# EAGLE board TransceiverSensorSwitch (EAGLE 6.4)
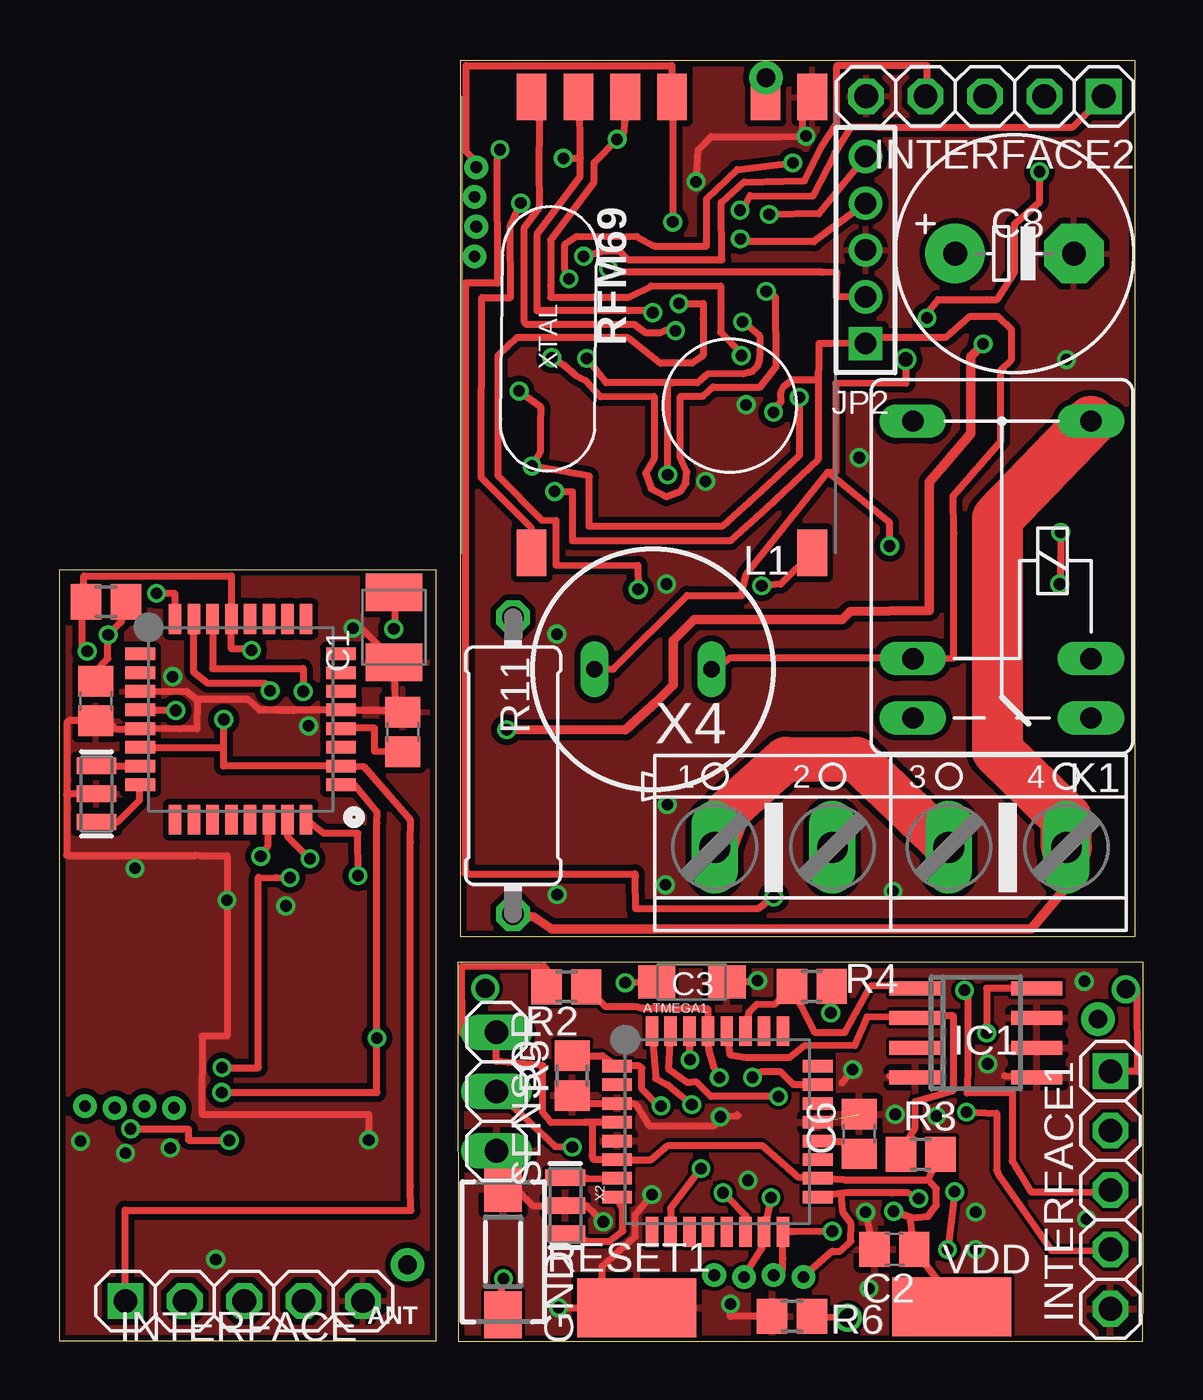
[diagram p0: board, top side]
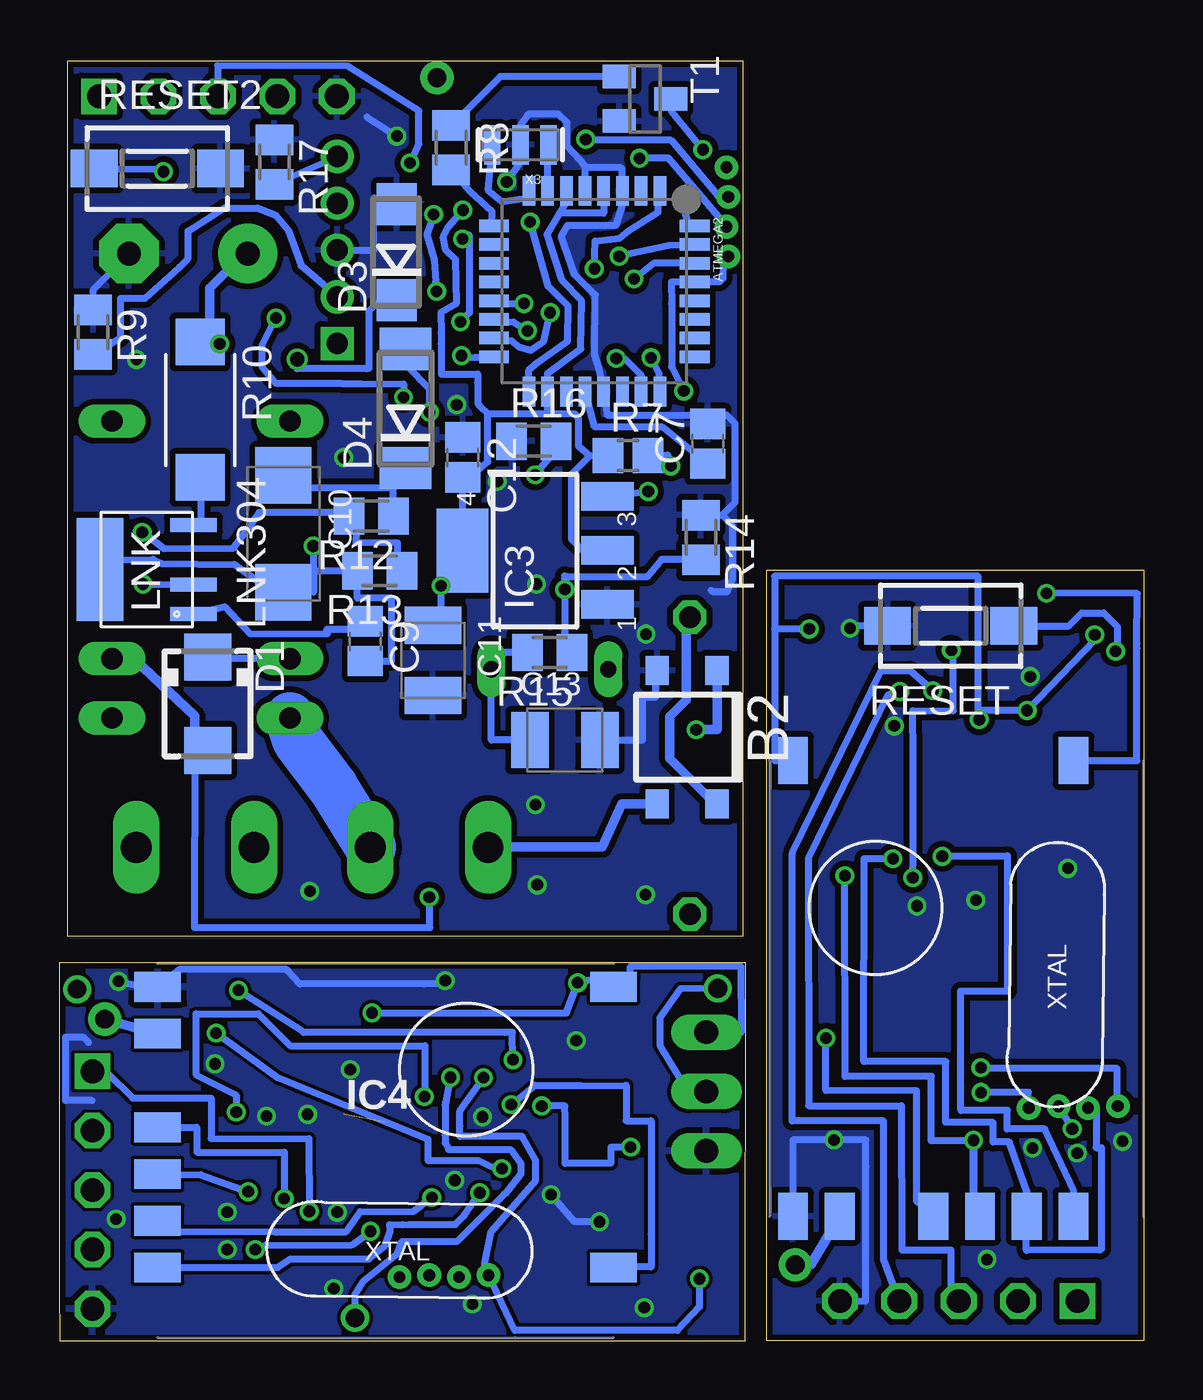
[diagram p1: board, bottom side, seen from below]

Size 46.36 x 54.77 mm. Coordinates in mm from the lower left corner, seen from the top.
Outline: 0,0.01 16.13,0.01 16.13,32.99 0,32.99 0,0.01
Outline: 17.06,0 46.34,0 46.35,2.34 46.36,15.39 46.35,16.2 17.04,16.2 17.06,0
Outline: 17.14,17.31 46.02,17.31 46.02,54.77 17.14,54.77 17.14,17.31
Copper layers (1*16): Top 0.035mm / dielectric 1.5mm / Bottom 0.035mm
Design rules "ITEADstudio_DRC": minimum track width 6mil, minimum drill 12mil, track to track 6mil, track to pad 6mil, pad to pad 6mil, via to via 6mil, smd to smd 0mil, copper to edge 10mil, drill to drill 10mil, minimum pad ring 10mil, minimum via ring 6mil, stop-mask expansion 2mil, vias tented up to drill 100mil, thermal gap 10mil
Net classes: 1 power: width 0.381 mm, clearance 0.254 mm; 2 220V: width 0.381 mm, clearance 0.508 mm

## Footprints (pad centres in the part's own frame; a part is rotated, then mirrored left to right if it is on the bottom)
TQFP32-08 = smd 1.27 x 0.533: 1 -4.293,2.8; 2 -4.293,2; 3 -4.293,1.2; 4 -4.293,0.4; 5 -4.293,-0.4; 6 -4.293,-1.2; 7 -4.293,-2; 8 -4.293,-2.8; 17 4.293,-2.8; 18 4.293,-2; 19 4.293,-1.2; 20 4.293,-0.4; 21 4.293,0.4; 22 4.293,1.2; 23 4.293,2; 24 4.293,2.8 | smd 0.533 x 1.27: 9 -2.8,-4.293; 10 -2,-4.293; 11 -1.2,-4.293; 12 -0.4,-4.293; 13 0.4,-4.293; 14 1.2,-4.293; 15 2,-4.293; 16 2.8,-4.293; 25 2.8,4.293; 26 2,4.293; 27 1.2,4.293; 28 0.4,4.293; 29 -0.4,4.293; 30 -1.2,4.293; 31 -2,4.293; 32 -2.8,4.293
TO-269AA = smd 1 x 1.25: + -1.28,-2.855; - 1.28,-2.855; AC1 -1.28,2.855; AC2 1.28,2.855
SMC_B = smd 1.6 x 2.4: + -1.5,0; - 1.5,0
C2012 = smd 1.3 x 1.5: 1 -0.85,0; 2 0.85,0
SMC_A = smd 1.6 x 1.4: + -1.5,0; - 1.5,0
E5-10,5 = drill 1.016 pad 2.54: + -2.54,0 | drill 1.016 pad 2.54 octagon: - 2.54,0
SMC_C = smd 2.4 x 2.4: + -2.5,0; - 2.5,0
SMA = smd 2 x 2: A 2,0; C -2,0
DO214AC = smd 1.8 x 1.7: A 2.05,0; C -2.05,0
DO214AA = smd 1.8 x 2.2: A 2.55,0; C -2.55,0
SMD2,54-5,08 = smd 2.54 x 5.08: 1 0,0
SO08 = smd 0.6 x 2.2: 1 -1.905,-2.6; 2 -0.635,-2.6; 3 0.635,-2.6; 4 1.905,-2.6; 5 1.905,2.6; 6 0.635,2.6; 7 -0.635,2.6; 8 -1.905,2.6
SOT223 = smd 1.219 x 2.235: 1 -2.311,-3.099; 2 0,-3.099; 3 2.311,-3.099 | smd 3.6 x 2.2: 4 0,3.099
RFM69W-MINPADS = smd 2 x 1.27: ANA 8,-5; DIO0 -11.5,5; GND 8,-7; MISO 8,1; MOSI 8,3; NSS 8,5; SCK 8,-1; VDD -11.5,-7
1X05-S = drill 1.016 square: 1 -5.08,0 | drill 1.016 octagon: 2 -2.54,0; 3 0,0; 4 2.54,0; 5 5.08,0
1X05M = drill 0.914 square: 1 -4,0 | drill 0.914: 2 -2,0; 3 0,0; 4 2,0; 5 4,0
FRS1B = drill 0.914 long: 1 0,3.81; 2 0,-3.81; O -2.54,-3.81; P 10.16,3.81; P@ 10.16,-3.81; S -2.54,3.81
BS11 = drill 0.7 long: 1 -2.5,0; 2 2.5,0
SO-8C = smd 0.6 x 2: BP -1.905,-2; D 1.905,-2; FB -0.635,-2 | smd 4.41 x 2: S 0,2
R2012 = smd 1.3 x 1.5: 1 -0.85,0; 2 0.85,0
M2012 = smd 1.3 x 1.6: 1 -0.95,0; 2 0.95,0
R2512W = smd 2 x 2.1: 1 -2.896,0; 2 2.896,0
0411/12 = drill 0.914 octagon: 1 -6.35,0; 2 6.35,0
DTSM-3 = smd 2 x 1.6: 1 -2.7,0; 2 2.7,0
1X03 = drill 1.016 long: 1 -2.54,0; 2 0,0; 3 2.54,0
SOT23 = smd 1 x 1.4: 1 -0.95,-1.1; 2 0.95,-1.1; 3 0,1.1
RFM12B-ANTENNA = drill 0.8 pad 1.422: P$1 0,0
AVRHEADER = drill 0.5: CLK 2.54,0; MISO 1.27,0.07; MOSI 0,0; VPP -1.27,0.072
RESONATOR-SMD = smd 0.7 x 1.7: 1 -1.2,0; 2 0,0; 3 1.2,0
AK500/4 = drill 1.321 long: 1 -7.518,0; 2 -2.489,0; 3 2.489,0; 4 7.518,0

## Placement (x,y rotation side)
ATMEGA1  ATMega-328  [TQFP32-08]  28.15,8.96 0 top
ATMEGA2  ATMega-328  [TQFP32-08]  23.49,44.91 270 bottom
ATMEGA328  ATMega-328  [TQFP32-08]  7.76,26.6 0 top
B2  RECT  [TO-269AA]  19.52,25.83 180 bottom
C1  100uF  [SMC_B]  14.32,30.53 90 top
C2  100nF  [C2012]  35.72,3.93 180 top
C3  100uF  [SMC_A]  27.06,15.36 0 top
C4  0.1  [C2012]  1.56,27.38 270 top
C5  0.1  [C2012]  14.69,26.05 90 top
C6  0.1  [C2012]  34.22,8.86 90 top
C7  0.1  [C2012]  18.64,38.39 90 bottom
C8  3,3uF  [E5-10,5]  40.86,46.52 0 top
C9  100nF  [C2012]  33.29,29.94 270 bottom
C10  22uF / 16 V  [SMC_C]  36.79,34.53 270 bottom
C11  100uF  [SMC_B]  30.39,29.12 270 bottom
C12  100nF  [C2012]  29.12,37.8 270 bottom
C13  100uF  [SMC_B]  24.75,25.71 0 bottom
D1  MBRA340T3  [SMA]  40.03,27.26 270 bottom
D3  ES1D  [DO214AC]  31.94,46.58 90 bottom
D4  1N4007GP  [DO214AA]  31.57,39.89 90 bottom
GND  [SMD2,54-5,08]  24.7,1.42 90 top
IC1  LM75AD  [SO08]  39.2,13.18 270 top
IC3  MC33269ST-3.3T3  [SOT223]  26.03,33.82 90 bottom
IC4  RFM69  [RFM69W-MINPADS]  34.17,8.15 180 bottom
INTERFACE  [1X05-S]  7.91,1.71 0 top
INTERFACE1  [1X05-S]  44.96,6.46 270 top
INTERFACE2  [1X05-S]  39.59,53.25 180 top
JP2  [1X05M]  34.49,46.67 90 top
K1  FRS1B  [FRS1B]  40.32,29.19 90 top
L1  680uH  [BS11]  25.4,28.74 0 top
LNK  LNK304  [SO-8C]  42.63,33.01 90 bottom
R1  10k  [R2012]  2,31.63 180 top
R2  10k  [R2012]  21.69,15.16 0 top
R3  10k  [R2012]  36.84,7.99 0 top
R4  10k  [R2012]  32.19,15.17 0 top
R5  10k  [R2012]  21.94,11.35 90 top
R6  10k  [R2012]  31.34,1.06 0 top
R7  10k  [R2012]  22.05,37.88 0 bottom
R8  1 K  [M2012]  29.62,51.05 90 bottom
R9  10K  [M2012]  44.93,43.16 270 bottom
R10  100  [R2512W]  40.35,39.85 270 bottom
R11  8,2  [0411/12]  19.41,24.62 90 top
R12  3.9 k  [M2012]  33.04,35.29 180 bottom
R13  2,05 k  [M2012]  32.68,32.95 180 bottom
R14  560  [M2012]  18.94,34.38 270 bottom
R15  470  [M2012]  25.4,29.46 180 bottom
R16  20K  [M2012]  26.09,38.5 0 bottom
R17  10K  [M2012]  37.17,50.44 270 bottom
RESET  RESET  [DTSM-3]  8.25,30.6 180 bottom
RESET1  [DTSM-3]  18.99,3.82 90 top
RESET2  RESET  [DTSM-3]  42.18,50.16 0 bottom
RFM69  RFM69  [RFM69W-MINPADS]  25.2,45.22 90 top
SENSOR  [1X03]  18.7,10.68 270 top
T1  BC846  [SOT23]  21.33,53.14 270 bottom
U$1  RFM12B_ANTENNA  [RFM12B-ANTENNA]  14.9,3.26 0 top
U$2  AVRHEADERDIP  [AVRHEADER]  2.38,9.97 0 top
U$3  RFM12B_ANTENNA  [RFM12B-ANTENNA]  44.43,13.77 0 top
U$4  AVRHEADERDIP  [AVRHEADER]  29.28,2.74 0 top
U$5  RFM69  [RFM69W-MINPADS]  8,13.33 270 bottom
U$6  RFM12B_ANTENNA  [RFM12B-ANTENNA]  30.22,54.04 0 top
U$7  AVRHEADERDIP  [AVRHEADER]  17.84,47.67 90 top
VDD  [SMD2,54-5,08]  38.17,1.47 90 top
X1  16 MHz  [RESONATOR-SMD]  1.6,23.41 270 top
X2  16 MHz  [RESONATOR-SMD]  21.65,5.8 270 top
X3  16 MHz  [RESONATOR-SMD]  26.66,51.17 180 bottom
X4  [AK500/4]  35.56,21.12 0 top

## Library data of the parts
ATMEGA1 ATMEGA2 ATMEGA328 IC4 RFM69 U$1 U$3 U$5 U$6 = LowPowerLab
B2 = rectifier
C1-C13 R1-R17 = resistor
D1 D3 D4 = diode
GND VDD = wirepad
IC1 = i2c
IC3 = linear
INTERFACE INTERFACE1 INTERFACE2 JP2 = pinhead-2
K1 = relay; OC_FARNELL: unknown; OC_NEWARK: unknown
L1 = inductor-neosid; OC_FARNELL: unknown; OC_NEWARK: unknown
LNK = powerint
RESET RESET1 RESET2 = switch-tact
SENSOR = pinhead
T1 = transistor
U$2 U$4 U$7 = RemoteHome
X1-X3 = SparkFun
X4 = con-ptr500; OC_FARNELL: unknown; OC_NEWARK: unknown

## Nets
5V: C13.+ D1.C D4.A IC3.3 JP2.1 K1.1 L1.2 R15.2
A0: ATMEGA328.23
A1: ATMEGA328.24
A2: ATMEGA328.25
A3: ATMEGA328.26
A4: ATMEGA1.22
A4_SDA: ATMEGA328.27
A4_SDA1: ATMEGA1.27 IC1.1 R4.1
A4_SDA2: ATMEGA2.27
A5: ATMEGA1.19
A5_SCL: ATMEGA328.28
A5_SCL1: ATMEGA1.28 IC1.2 R3.1
A5_SCL2: ATMEGA2.28
A6: ATMEGA328.19
A7: ATMEGA328.22
A8: ATMEGA1.26
A9: ATMEGA1.25
A10: ATMEGA1.24
A11: ATMEGA1.23 R6.2
A12: ATMEGA2.22
A13: ATMEGA2.19
A14: ATMEGA2.26
A15: ATMEGA2.25
A16: ATMEGA2.24 JP2.5 R17.2
A17: ATMEGA2.23 JP2.4 R16.2
AREF: ATMEGA328.20 C5.1
AREF1: ATMEGA1.20 C6.1
AREF2: ATMEGA2.20 C7.1
D0_RX: ATMEGA328.30 INTERFACE.3
D0_RX1: ATMEGA1.30 INTERFACE1.3
D0_RX2: ATMEGA2.30 INTERFACE2.3
D1: ATMEGA1.13
D1_TX: ATMEGA328.31 INTERFACE.4
D1_TX1: ATMEGA1.31 INTERFACE1.4
D1_TX2: ATMEGA2.31 INTERFACE2.4
D2: ATMEGA328.32 U$5.DIO0
D3: ATMEGA328.1
D4: ATMEGA328.2
D5: ATMEGA328.9
D6: ATMEGA328.10
D7: ATMEGA328.11
D8: ATMEGA328.12
D9: ATMEGA328.13
D10: ATMEGA1.12
D10_SS: ATMEGA328.14 U$5.NSS
D10_SS1: ATMEGA1.14 IC4.NSS
D10_SS2: ATMEGA2.14 RFM69.NSS
D11: ATMEGA1.11
D11_MOSI: ATMEGA328.15 U$2.MOSI U$5.MOSI
D11_MOSI1: ATMEGA1.15 IC4.MOSI U$4.MOSI
D11_MOSI2: ATMEGA2.15 RFM69.MOSI U$7.MOSI
D12: ATMEGA1.10 IC1.8
D12_MISO: ATMEGA328.16 U$2.MISO U$5.MISO
D12_MISO1: ATMEGA1.16 IC4.MISO U$4.MISO
D12_MISO2: ATMEGA2.16 RFM69.MISO U$7.MISO
D13: ATMEGA1.9
D13_SCK: ATMEGA328.17 U$2.CLK U$5.SCK
D13_SCK1: ATMEGA1.17 IC4.SCK U$4.CLK
D13_SCK2: ATMEGA2.17 RFM69.SCK U$7.CLK
D14: ATMEGA1.2
D15: ATMEGA1.1 R5.2 SENSOR.2
D16: ATMEGA1.32 IC4.DIO0
D17: ATMEGA2.13 R14.2 R15.1
D18: ATMEGA2.12
D19: ATMEGA2.11
D20: ATMEGA2.10
D21: ATMEGA2.9 R8.1
D22: ATMEGA2.2
D23: ATMEGA2.1 JP2.2 R9.2
D24: ATMEGA2.32 RFM69.DIO0
FB: LNK.FB R12.2 R13.1
GND [power]: ATMEGA328.3 ATMEGA328.5 ATMEGA328.21 C1.+ C4.2 C5.2 INTERFACE.5 RESET.2 U$5.GND X1.2
GND1: ATMEGA1.3 ATMEGA1.5 ATMEGA1.21 C2.2 C3.- C6.2 GND.1 IC1.4 IC1.5 IC1.6 IC1.7 IC4.GND INTERFACE1.5 R5.1 R6.1 RESET1.2 SENSOR.3 X2.2
GND2 [power]: ATMEGA2.3 ATMEGA2.5 ATMEGA2.21 B2.- C7.2 C8.- C11.- C12.1 C13.- D3.A IC3.1 INTERFACE2.5 JP2.3 R9.1 R14.1 R16.1 R17.1 RESET2.2 RFM69.GND T1.2 X3.2
N$1: ATMEGA328.7 X1.1
N$2: ATMEGA1.7 X2.1
N$3: U$1.P$1 U$5.ANA
N$4: ATMEGA1.8 X2.3
N$5: IC4.ANA U$3.P$1
N$6: ATMEGA2.7 X3.1
N$7: ATMEGA2.8 X3.3
N$8: RFM69.ANA U$6.P$1
N$9 [220V]: K1.P@ R11.1 X4.4
N$10 [220V]: B2.AC2 X4.1 X4.3
N$11 [220V]: K1.S X4.2
N$12: D1.A K1.2 T1.3
N$13 [220V]: LNK.D R10.2
N$14 [220V]: B2.+ C8.+ R10.1
N$15 [220V]: B2.AC1 R11.2
N$16: R8.2 T1.1
N$17: C9.2 C10.- D3.C L1.1 LNK.S R13.2
N$18: C9.1 LNK.BP
N$19 [220V]: K1.P
N$20: C10.+ D4.C R12.1
N$21: ATMEGA328.8 X1.3
N$22 [220V]: K1.O
RST: ATMEGA328.29 R1.2 RESET.1 U$2.VPP
RST1: ATMEGA1.29 R2.2 RESET1.1 U$4.VPP
RST2: ATMEGA2.29 R7.2 RESET2.1 U$7.VPP
VCC: ATMEGA328.4 ATMEGA328.6 ATMEGA328.18 C1.- C4.1 INTERFACE.1 R1.1 U$5.VDD
VCC1: ATMEGA1.4 ATMEGA1.6 ATMEGA1.18 C2.1 C3.+ IC4.VDD INTERFACE1.1 R2.1 R3.2 R4.2 SENSOR.1 VDD.1
VCC2: ATMEGA2.4 ATMEGA2.6 ATMEGA2.18 C11.+ C12.2 IC3.2 IC3.4 INTERFACE2.1 R7.1 RFM69.VDD

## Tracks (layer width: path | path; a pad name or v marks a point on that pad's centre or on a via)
5V  (via drill 0.5)
  Top 0.305: L1.2 28.03,28.74 28.03,28.75 28.03,28.69 28.7,29.23 35.78,29.24 K1.1 38.26,29.22 38.26,34.54 38.23,36.16 40.26,38.5 40.26,41.53 40.73,41.99 40.73,43.26 40.17,43.82 38.92,43.82 37.91,42.93 34.87,42.93 JP2.1 33.48,42.68 33.04,42.67 32.49,42.67 32.49,41.61 32.47,41.45 | 32.47,41.45 32.46,37.71 30.23,35.62 28.71,34.22 21.96,34.22 21.96,34.93 21.96,36.32 21.55,36.32 v21.19,36.34 | v30.54,39.73 30.87,40.19 30.86,40.57 30.99,40.85 31.36,41.12 32.48,41.12 32.47,41.45
  Bottom 0.305: K1.1 39.96,29.19 D1.C | 22.82,36.24 IC3.3 | IC3.3 22.57,36.13 | v21.19,36.34 22.91,36.11 IC3.3 | R15.2 27.9,29.46 L1.2 27.9,25.71 C13.+ | D4.A 31.57,41.77 30.54,40.74 v30.54,39.73
A4_SDA1
  Top 0.305: 29.3,13.73 29.33,13.28 | 29.33,13.28 ATMEGA1.27 | 29.33,13.28 29.51,14.08 29.85,14.42 30.59,14.4 R4.1 31.34,15.15 31.42,14.97 32.34,13.19 33.58,13.19 34.7,15.19 35.61,15.19 IC1.1
A5_SCL1
  Top 0.305: ATMEGA1.28 28.56,13.24 28.7,12.23 29.36,12.12 31.22,12.12 31.89,12.65 34.03,12.63 34.55,13.88 IC1.2 35.9,13.91 38.25,13.91 38.25,10.73 36.6,10.24 36.6,9.13 35.98,8.09 R3.1
A11  (via drill 0.5, 0.8)
  Top 0.305: ATMEGA1.23 31.41,10.96 30.86,11.51 30.01,11.51 v29.65,11.28 | R6.2 v33.73,0.99
  Bottom 0.305: v29.65,11.28 29.86,10.22 29.87,10.09 29.87,8.92 29.88,8.81 29.88,8.47 29.72,8.2 27.07,8.2 26.63,7.6 26.63,7.15 27.33,6.28 27.35,6.28 29.39,4.25 31.75,4.24 31.93,3.7 33.37,2.56 33.73,2 v33.73,0.99
A16  (via drill 0.5)
  Top 0.305: JP2.5 32.49,48.23 v30.37,48.19 | v21.07,42.06 21.57,41.74 22.06,41.32 22.52,41.09 23.15,40.4 25.45,40.42 25.45,37.74 25.08,37.13 25.32,36.46 25.97,36.12 26.59,36.37 26.8,36.69 26.84,37.18 26.57,37.8 26.57,40.42 27.53,40.42 27.96,40.82 29.99,40.82 30.66,41.68 30.64,44.65 v30.24,44.9
  Bottom 0.305: v30.37,48.19 30.66,47.33 30.35,46.24 30.27,45.3 v30.24,44.9 | ATMEGA2.24 20.72,41.4 v21.07,42.06 | R17.2 JP2.5
A17  (via drill 0.5)
  Top 0.305: JP2.4 33.08,47.63 32.27,47.03 29.19,47.03 v29.13,47.15 | v29.22,43.6 29.29,43.57 29.95,43.01 29.96,42.27 29.95,41.96 29.86,41.71 29.64,41.48 29.53,41.44 29.26,41.37 27.75,41.38 27.3,40.99 26.27,40.99 | 26.27,40.99 23.39,40.99 v22.56,42.04 | v26.02,37.06 26.02,40.99 26.27,40.99
  Bottom 0.305: v29.13,47.15 29.16,47.31 28.85,47.31 28.83,43.99 v29.22,43.6 | v22.56,42.04 22.18,42.01 21.49,41.33 ATMEGA2.23 | R16.2 25.08,38.18 v26.02,37.06
AREF
  Top 0.305: C5.1 13.49,25.22 13.49,26.22 12.63,26.22 ATMEGA328.20
AREF1
  Top 0.305: ATMEGA1.20 32.49,8.51 33.48,8.51 34.08,7.91 C6.1
AREF2
  Bottom 0.305: 23.91,40.34 ATMEGA2.20 23.47,39.1 20.66,39.1 20.57,39.09 C7.1
D0_RX  (via drill 0.5)
  Top 0.305: ATMEGA328.30 6.56,28.76 10.44,28.78 v10.44,27.79
  Bottom 0.305: v10.44,27.79 10.96,27.61 14.34,20.66 14.32,10.06 10.36,10.06 10.34,3.89 8.23,3.89 8.22,1.86 INTERFACE.3
D0_RX1  (via drill 0.5)
  Top 0.305: ATMEGA1.30 26.95,12.51 v26.98,12.03 | v38.71,15.01 38.86,15.01 38.85,14.23 38.85,12.05 38.86,11.93 38.83,10.61 40.76,10.64 40.75,7.71 41.58,6.37 | 42.05,6.37 41.58,6.37 | 41.58,6.37 44.23,6.39 INTERFACE1.3
  Bottom 0.305: v26.98,12.03 27,13.21 27.31,13.2 35.93,13.2 36.02,13.29 v38.71,15.01
D0_RX2  (via drill 0.5)
  Top 0.305: v21.8,45.43 21.62,45.89 21.62,46.92 22.13,47.26 24.7,47.25 25.44,46.84 27.69,46.84 27.69,48.86 28.99,50.11 30.71,50.32 v31.38,50.4
  Bottom 0.305: ATMEGA2.30 20.96,46.11 v21.8,45.43 | v31.38,50.4 30.99,51.22 31,52.63 34.05,54.54 39.6,54.56 INTERFACE2.3
D1_TX  (via drill 0.5)
  Top 0.305: v9.02,27.82 8.81,28.13 6.37,28.13 5.76,28.59 ATMEGA328.31
  Bottom 0.305: INTERFACE.4 10.52,1.86 11.12,3.49 11.12,9.42 15.03,9.42 15.03,20.88 11.21,28.69 10,28.69 v9.02,27.82
D1_TX1  (via drill 0.5)
  Top 0.305: v30.76,10.46 27.87,10.46 27.25,11.08 26.89,11.05 26.07,11.62 26.16,13.24 ATMEGA1.31 | v38.8,9.79 40.09,9.75 40.09,7.3 40.17,7.14 42.45,3.86 44.27,3.89 INTERFACE1.4
  Bottom 0.305: v30.76,10.46 30.76,10.51 30.75,10.52 30.74,12.63 36.49,12.63 37.86,14 40.52,14 40.51,11.38 38.81,10.53 v38.8,9.79
D1_TX2  (via drill 0.5)
  Top 0.305: INTERFACE2.4 37.13,53.46 37.13,54.55 33.26,54.56 33.25,52.1 32.61,51.11 31.88,49.64 29.28,49.58 28.31,48.71 28.34,46.26 24.31,46.27 23.95,46.64 23.59,46.64 23.28,46.64 23.16,46.6 v22.43,46.4
  Bottom 0.305: ATMEGA2.31 20.3,46.86 v22.43,46.4
D2  (via drill 0.5)
  Top 0.305: v4.16,31.99 4.94,31.99 ATMEGA328.32
  Bottom 0.305: v4.16,31.99 0.28,31.98 0.29,29.86 0.29,29.64 0.29,24.83 U$5.DIO0
D10_SS  (via drill 0.5)
  Top 0.305: v8.62,20.74 8.94,21.2 ATMEGA328.14
  Bottom 0.305: U$5.NSS 3,6.44 4.23,9.07 5.84,9.08 5.84,9.18 5.84,9.87 7.82,9.86 7.82,9.97 7.83,14.97 5.83,14.98 5.83,20.76 5.84,20.74 6.62,20.74 v8.62,20.74
D10_SS1  (via drill 0.5)
  Top 0.305: v28.39,6.34 28.57,6.17 29.37,5.37 29.39,4.71 ATMEGA1.14
  Bottom 0.305: IC4.NSS 37.03,3.15 36.49,3.51 33.13,3.51 32.44,4.08 32.23,4.7 32.25,4.99 31.71,4.98 31.42,4.99 31.11,4.98 29.44,4.98 29.07,5.35 v28.39,6.34
D10_SS2  (via drill 0.5)
  Top 0.305: RFM69.NSS 20.53,52.23 20.52,50 20.53,48.81 20.53,48.5 19.88,47.61 19.88,43.61 19.98,43.49 24.59,43.49 25.09,43.13 25.69,43.13 26.25,43.37 v26.36,43.22
  Bottom 0.305: ATMEGA2.14 27.76,43.68 26.96,43.59 v26.36,43.22
D11_MOSI  (via drill 0.5)
  Top 0.305: ATMEGA328.15 9.76,21.59 v10.73,20.63
  Bottom 0.305: v10.73,20.63 10.91,20.65 11.95,20.64 11.96,11.96 8.47,11.96 8.47,9.36 6.44,9.35 6.44,8.52 5.75,8.52 5,6.41 U$5.MOSI 5.02,3.88 1.86,3.9 1.81,3.93 1.81,8.28 2.04,8.28 2.04,9.98 2.02,9.98 U$2.MOSI
D11_MOSI1  (via drill 0.5)
  Top 0.305: v30.44,6.14 30.13,4.69 ATMEGA1.15 30.05,3.97 U$4.MOSI
  Bottom 0.305: IC4.MOSI 41.4,4.7 37.18,4.68 34.1,4.68 33.51,5.54 31.24,5.54 v30.44,6.14
D11_MOSI2  (via drill 0.5)
  Top 0.305: v25.39,44 25.22,44.08 24.35,44.07 23.32,44.07 20.44,44.07 20.44,47.35 22.28,49.8 22.28,50.7 | 22.28,50.7 22.27,53.18 RFM69.MOSI | v21.56,50.6 22.3,50.6 22.28,50.7
  Bottom 0.305: ATMEGA2.15 27.02,42.79 26.76,42.55 26.2,42.38 25.66,42.76 v25.39,44 | U$7.MOSI 19.05,49.09 20.33,50.6 21.68,50.6 v21.56,50.6
D12  (via drill 0.5)
  Top 0.305: IC1.8 39.66,15.09 v39.67,13.17 | v27.45,7.38 26.13,5.69 26.15,5.64 ATMEGA1.10
  Bottom 0.305: v39.67,13.17 39.2,12.84 37,11.25 30.61,8.64 30.61,7.73 28.44,7.73 27.39,7.22 v27.45,7.38
D12_MISO  (via drill 0.5)
  Top 0.305: v12.78,19.91 12.77,21.72 11.32,21.72 ATMEGA328.16 | v3.06,9.08 5.53,9.08 5.53,8.59 v7.28,8.59
  Bottom 0.305: U$5.MISO 7.29,5.47 | 7.29,5.47 7.29,8.57 9.1,8.57 9.08,11.33 12.77,11.32 v12.78,19.91 | U$2.MISO 3.62,10.04 v3.06,9.08 | v7.28,8.59 7.28,6.36 7.29,5.47
D12_MISO1  (via drill 0.5)
  Top 0.305: v38.29,6.39 v37.99,3.91 | v33.06,4.69 31.43,4.68 ATMEGA1.16 | U$4.MISO 30.93,3.07 30.95,3.53 ATMEGA1.16 | ATMEGA1.16
  Bottom 0.305: IC4.MISO 40.31,7.11 v38.29,6.39 | v37.99,3.91 37.71,3.92 37.56,4.1 33.84,4.13 v33.06,4.69
D12_MISO2  (via drill 0.5)
  Top 0.305: RFM69.MISO 24.18,52.13 24.16,51.71 24.08,51.59 23.73,51.25 v23.86,51.41 22.88,50.41 22.88,49.6 21.01,47.11 21.01,45.16 21.01,44.65 24.36,44.65 25.31,45.14 28.28,45.14 28.28,43.16 29.17,42.27 v29.17,42.15
  Bottom 0.305: v29.17,42.15 29.18,42.08 28.6,42.08 27.66,42.08 ATMEGA2.16 | v23.86,51.41 23.82,51.37 20.21,51.37 18.2,48.97 17.97,48.94 U$7.MISO
D13_SCK  (via drill 0.5)
  Top 0.305: ATMEGA328.17 12.62,23.8 13.6,22.62 13.6,22.59 13.59,22.18 v13.59,12.96 13.59,10.63 v6.96,10.63
  Bottom 0.305: U$5.SCK 9.71,5.98 9.71,10.7 13.59,10.72 v13.59,12.96 | U$2.CLK 4.93,10.64 v6.96,10.63
D13_SCK1  (via drill 0.5)
  Top 0.305: v36.76,6.1 36.28,6.35 35.62,6.34 33.67,6.35 33.45,6.31 | 33.45,6.31 ATMEGA1.17 | U$4.CLK 33.06,3.85 33.4,3.85 33.86,4.28 33.87,5.01 33.8,5.12 33.51,5.53 33.45,6.31
  Bottom 0.305: IC4.SCK 40.5,9.15 40.49,8.07 36.75,8.08 v36.76,6.1
D13_SCK2  (via drill 0.5)
  Top 0.305: v26.24,47.87 26.26,47.96 26.26,51.94 26.26,53.18 RFM69.SCK | 26.4,53.41 RFM69.SCK | U$7.CLK 17.69,50.6 17.39,50.89 17.41,50.89 17.41,54.56 26.2,54.56 RFM69.SCK
  Bottom 0.305: ATMEGA2.17 26.29,41.54 25.89,41.88 24.63,42.77 24.62,44.28 25.47,45.12 v26.24,47.87
D15  (via drill 0.5, 0.8)
  Top 0.305: R5.2 23.23,12.2 ATMEGA1.1 24.8,11.77 24.92,11.68 24.92,10.79 25.68,9.99 v25.74,10.06 | SENSOR.2 21.2,8.33 v21.94,8.29
  Bottom 0.305: v25.74,10.06 24.75,10.06 24.74,9.57 24.74,7.6 22.79,7.6 22.79,8.29 v21.94,8.29 | v18.22,15.09 19.82,15.07 20.69,13.83 20.69,12.66 19.54,10.74 18.77,10.74
  Bottom 0.406: 18.77,10.74 SENSOR.2
D16  (via drill 0.5)
  Top 0.305: ATMEGA1.32 25.5,11.55 25.51,11.24 26.05,10.94 v27.05,10.11
  Bottom 0.305: v27.05,10.11 26.02,10.94 24.07,10.94 24.06,10.93 22.13,10.95 22.13,9.43 21.07,9.43 21.06,4.57 21.06,3.17 21.78,3.17 IC4.DIO0
D17  (via drill 0.5)
  Top 0.305: v26.5,44.38 27.55,44.38 27.54,43.75 27.54,42.17 27.06,41.83 25.71,41.83 24.33,42.92 19.56,42.92 18.77,42.17 18.77,37.01 20.65,35.11 21.24,35.11 21.24,33.19 24.75,33.19 v24.76,32.15
  Bottom 0.305: ATMEGA2.13 27.53,44.38 v26.5,44.38 | R14.2 18.9,33.43 18.89,33.43 20.62,33.43 21.24,32.69 24.6,32.68 24.76,32.73 24.76,32.64 v24.76,32.15 24.76,30.32 24.76,29.47 24.58,29.47 24.82,29.46 R15.1
D21
  Bottom 0.305: ATMEGA2.9 27.88,47.71 27.87,48.31 28.78,49.16 R8.1
D23  (via drill 0.5)
  Top 0.305: JP2.2 33.25,44.65 33.26,45.6 33.27,45.71 32.63,45.72 23.83,45.73 v23.49,45.88
  Bottom 0.305: v23.49,45.88 23.45,47.07 23.47,47.05 22.4,47.18 22.01,47.5 20.77,48.28 20.77,48.57 20.77,49.12 ATMEGA2.1 | R9.2 43.75,42.93 43.75,44.47 43.75,44.61 42.71,44.61 41.23,45.94 40.86,46.31 40.86,47.48 39.31,48.47 37.89,48.47 37.11,48.16 36.58,47.51 36.03,45.99 JP2.2
D24  (via drill 0.5)
  Top 0.305: v19.74,48.68 19.3,47.71 19.31,44.64 18.07,44.64 18.05,36.94 20.2,34.77 RFM69.DIO0 20.22,33.73
  Bottom 0.305: v19.74,48.68 19.48,47.76 19.25,47.68 19.23,47.71 ATMEGA2.32
FB  (via drill 0.5)
  Top 0.305: v42.83,34.6 42.83,33.51 v42.79,32.38
  Bottom 0.305: v42.83,34.6 41.88,33.88 38.95,33.91 37.83,35.45 34.79,35.45 34.12,35.47 R12.2 33.8,35.22 33.65,34.63 33.68,34.16 31.91,34.14 31.94,32.6 R13.1 | v42.79,32.38 40.64,32.35 LNK.FB
GND  (via drill 0.5)
  Top 0.305: 4.03,26.22 ATMEGA328.5 | ATMEGA328.3 5.44,27.8 5.9,27.45 | 5.9,27.45 5.88,26.2 5.16,26.18 ATMEGA328.5 | 8.57,26.99 ATMEGA328.21 12.63,26.98 13.05,26.98 14.55,26.98 C5.2 14.38,27.35 C1.+ 13.79,29.45 13.79,29.63 12.93,30.49 v12.56,30.49 | 8.57,26.99 8.09,27.44 5.9,27.45 | 10.03,26.96 8.57,26.99 | v13.24,8.6 13.22,8.45 13.24,9.69 6.11,9.7 6.11,13.04 7.18,13.04 7.18,20.76 6.12,20.76 6,20.77 5.82,20.79 5.82,20.77 0.32,20.78 0.32,23.37 | 0.35,23.43 X1.2 0.43,23.38 0.32,23.37 | 0.35,23.43 0.32,23.37 | ATMEGA328.5 2.43,26.19 2.09,26.53 C4.2 1.53,26.56 0.45,26.56 0.35,26.49 0.35,23.43
  Bottom 0.305: 14.5,5.33 U$5.GND 15,8.6 v13.24,8.6 11.88,8.6 11.88,7.46 11.9,1.71 INTERFACE.5 | RESET.2 12.46,30.6 v12.56,30.49
  other vias: 9.69,18.62 4.75,8.26 0.91,8.55 2.84,8.04 6.7,3.49 7.18,18.86 3.24,20.22 4.85,28.42 10.67,26.32
  pour Bottom: 0.15,32.87 15.99,32.83 15.97,0.15 0.14,0.15 0.14,29.89
  pour Top: 15.97,32.87 15.99,29.9 15.99,0.15 0.16,0.15 0.15,32.89
GND1  (via drill 0.5)  (1 unrouted)
  Top 0.305: IC1.4 35.51,11.33 | 32.45,9.37 ATMEGA1.21 | GND.1 23.3,1.44 22.87,1.44 v21.36,1.43 23.24,1.43 23.24,1.98 23.22,3.2 24.64,4.48 24.62,5.4 v25.35,6.27 | IC1.5 40.44,11.33 40.42,11.35 | C3.- 28.71,15.38 v29.87,15.42 | R5.1 22.19,10.59 22.34,10.16 ATMEGA1.3 24.6,10.16 24.76,9.97 25.23,9.21 25.97,9.2 27.35,9.2 28.01,9.21 28.39,9.62 v28.27,9.59 29.03,9.64 28.99,9.68 | v23.27,5.11 22.54,5.8 X2.2 20.25,5.79 19.5,6.55 RESET1.2 | 18.68,6.55 SENSOR.3 | v34.49,5.51 34.73,4.27 C2.2 | v33.93,11.61 33.47,11.03 | R6.1 28.7,1.06 v28.71,1.59
  Top 0.406: RESET1.2 18.68,6.55
  Bottom 0.305: v43.84,15.39 42.9,15.15 IC4.GND 41.26,15.85 41.25,15.89 36.64,15.89 36.58,15.82 36.08,15.28 33.96,15.28 33.11,15.28 30.77,15.27 30.16,15.28 29.89,15.42 v29.87,15.42 | v23.27,5.11 24.35,5.11 v25.35,6.27 | 44.97,10.29 46.1,10.29 46.1,13.01 45.35,13.01 45.12,12.77
  other vias: 35.75,9.7 29.46,6.88 39.71,11.86 37.51,9.62 34.63,2.25 39.2,5.51 39.2,3.92 24.27,12.85 43.94,5.22
  pour Top: 17.26,16.05 46.23,16.03 46.16,0.18 17.26,0.22
  pour Bottom: 17.23,16.02 46.19,16.04 46.19,0.15 17.26,0.17
GND2  (via drill 0.5)
  Top 0.305: RFM69.GND 31.73,53.17 31.8,52.77 31.79,51.7 v31.94,51.55 30.85,51.52 27.89,51.52 27.32,50.94 v27.24,49.59
  Bottom 0.305: ATMEGA2.5 23.89,50.19 23.87,50.21 | 23.87,50.21 22.39,50.21 22.31,50.13 22.31,48.93 ATMEGA2.3 22.21,48.83 22.56,47.73 24.63,47.73 24.81,47.41 24.9,47.27 24.33,45.62 23.45,44.75 23.48,42.2 23.29,41.59 ATMEGA2.21 23.11,40.61 22.95,39.62 19.03,39.62 | 23.87,50.21 24.15,50.57 24.67,51.13 24.67,52.13 25.05,52.5 26.29,52.5 26.66,51.97 X3.2 26.66,50.43 v27.24,49.59 | D3.A 32.3,49.24 | 32.3,49.24 32.46,49.4 | 31.54,48.17 31.86,48.85 D3.A | R9.1 44.92,44.97 C8.- | 19.03,39.62 C7.2 | R14.1 18.03,35.33 | 18.03,35.33 17.61,34.9 17.61,32.56 17.81,32.04 18.43,32.04 18.51,32.12 | 19.03,39.62 17.84,39.62 17.48,39.26 17.48,35.88 18.03,35.33 | D3.A 31.96,49.13 | JP2.3 32.92,46.68 32.91,48.9 32.65,48.9 32.3,49.24 | C13.- 21.43,25.71 21.43,27.56 20.86,27.56 20.86,28.35 | 33.22,52.36 v31.94,51.55
  Bottom 0.406: B2.- 20.86,28.35 | R9.1 44.89,44.33
  other vias: 29.38,40.06 26.01,22.94 21.28,30.24 35.66,19.24 21.3,19.1 25.93,19.52 27.65,36.78 25.97,32.39 34.21,37.79 43.07,41.99
  pour Top: 17.27,54.61 45.9,54.61 45.9,17.44 17.27,17.44 17.27,54.54
  pour Bottom: 17.33,54.61 45.9,54.61 45.9,17.44 17.3,17.44 17.3,54.64
N$1
  Top 0.305: X1.1 ATMEGA328.7
N$2
  Top 0.305: X2.1 22.07,6.99 22.55,6.97 ATMEGA1.7
N$3
  Bottom 0.406: U$5.ANA 14.24,3.27 U$1.P$1
N$4
  Top 0.305: X2.3 22.66,4.26 23.55,4.26 24.1,4.71 24.1,5.62 23.85,6.15 ATMEGA1.8
N$5
  Bottom 0.406: IC4.ANA U$3.P$1
N$6
  Bottom 0.305: ATMEGA2.7 25.49,50.79 X3.1
N$7
  Bottom 0.305: X3.3 28.05,49.24 27.45,48.75 26.29,48.91 ATMEGA2.8
N$8
  Top 0.406: RFM69.ANA 30.27,53.19 U$6.P$1
N$9
  Top 0.406: R11.1 20.29,18.15 21.07,17.63 41.57,17.64 43.13,19.49 43.13,21.06 X4.4
  Top 2.184: X4.4 43.08,22.37 40.13,25.25 40.13,35.2 K1.P@
N$10
  Top 1.93: X4.1 28.6,22.67 31.06,24.88 34.09,24.9 X4.3
  Bottom 0.406: B2.AC2 22.32,22.98 23.15,21.13 28.02,21.13 X4.1
N$11
  Bottom 2.184: K1.S 36.19,25.72 34.68,23.71 X4.2
N$12  (via drill 0.5)
  Top 0.305: v30.56,18.99 | v30.56,18.99 29.89,18.5 24.65,18.5 24.63,19.79 | 24.63,19.79 24.63,19.95 | v18.85,50.97 18.74,50.68 18.71,50.42 18.72,45.32 18.74,45.25 17.36,45.25 17.36,19.98 24.63,19.98 24.63,19.79
  Bottom 0.305: D1.A 40,25.46 40.56,25.46 40.59,17.68 30.53,17.68 30.53,18.6 v30.56,18.99 | T1.3 20.2,52.6 v18.85,50.97
  Bottom 0.406: K1.2 43.17,29.17 40.58,26.74 40.58,26.05 D1.A
N$13
  Bottom 0.305: R10.2 40.31,34.9 LNK.D
N$14  (via drill 0.5)
  Top 0.406: v19.14,26.15 24.21,26.14 25.55,27.36 25.56,27.36 26.26,28.05 26.26,29.96 27.16,30.86 33.48,30.86 33.83,31.21 37.21,31.24 37.22,36.75 38.98,38.83 38.98,41.46 | 38.98,41.46 | 38.98,41.46 38.98,42.11 v39.51,42.66
  Bottom 0.305: R10.1 39.6,42.74 v39.51,42.66
  Bottom 0.406: C8.+ 38.46,46.52 39.93,45.04 39.93,43.14 R10.1 | B2.+ 18.24,26.15 v19.14,26.15
N$15
  Bottom 0.406: R11.2 19.56,30.86 19.56,27.42 20.27,26.71 20.27,24.92 18.27,22.9 18.3,22.72 B2.AC1
N$16
  Bottom 0.305: T1.1 27.52,54.09 R8.2
N$17  (via drill 0.5, 0.6)
  Top 0.305: v36.2,41.99 36.21,40.97 33.21,40.97 33.2,37.16 32.86,37.16 | 32.86,37.16 29.36,32.8 29.21,32.17 29.2,31.89 26.85,31.89 23.7,28.74 L1.1 | v35.51,34.01 35.51,35.01 32.86,37.16
  Bottom 0.305: LNK.S 44.02,33.41 42.32,33.43 42.42,33.42 42.01,33.27 38.9,33.23 37.14,31.96 C10.- | C10.- 35.88,32.96 R13.2 | R13.2 33.61,32.5 | D3.C 31.91,44.61 31.96,44.56 32.63,44.56 33.13,44.06 33.13,41.6 33.23,41.59 36.2,41.59 v36.2,41.99 | C9.2 32.16,29.09 32.16,31.78 33.63,31.78 R13.2 | v35.51,34.01 35.5,32.03 C10.-
N$18
  Bottom 0.305: LNK.BP 39.3,31.41 38.22,30.25 34.9,30.26 34.93,30.46 32.88,30.46 C9.1
N$20
  Bottom 0.305: R12.1 32.09,36.69 D4.C 32.1,37.48 32.1,36.48 35.76,36.48 35.76,36.58 C10.+
N$21
  Top 0.305: X1.3 2.5,22.21 3.44,23.15 3.44,23.77 ATMEGA328.8
RST  (via drill 0.5)
  Top 0.305: v6.96,11.7 8.51,11.7 8.51,19.84 9.29,19.82 v9.87,19.82 | v8.23,29.55 8.2,29.55 8.28,29.6 7.37,29.61 ATMEGA328.29 7.36,32.73 1.05,32.73 1.05,31.88 R1.2 0.98,31.42 0.98,29.48 v1.2,29.51
  Bottom 0.305: U$2.VPP 1.14,10.04 1.14,11.66 6.96,11.66 v6.96,11.7 | v9.87,19.82 9.87,20.77 9.87,25 9.88,26.97 8.14,26.95 8.14,29.27 v8.23,29.55 | RESET.1 3.21,30.6 2.65,31.15 1.72,31.15 1.13,30.56 1.13,29.41 v1.2,29.51
RST1  (via drill 0.5)
  Top 0.305: RESET1.1 18.99,1.16 18.91,1.24 18.91,2.08 v19,2.66 | v28.23,11.27 28.01,11.68 27.78,12.5 27.74,13.24 ATMEGA1.29 27.73,13.28 27.73,14.22 25.95,14.25 24.87,14.26 24.69,14.31 23.36,14.31 22.7,15 R2.2
  Bottom 0.305: v19,2.66 19,1.46 19.95,0.45 26.89,0.45 U$4.VPP 28.19,3.05 28.18,3.33 27.9,4.69 26,6.87 26,7.73 26.57,8.75 29.24,8.75 29.25,9.2 29.25,9.84 v28.23,11.27
RST2  (via drill 0.5)
  Top 0.305: v41.92,50.02 41.92,48.72 40.85,47.8 40.85,45.72 40.11,44.56 39.67,44.56 37.59,44.56 37.11,43.94 v37.11,43.76 | v31.66,40.37 31.66,37.89 29.95,36.3 28.35,34.85 22.66,34.85 22.67,36.99 v20.22,37.44 20.58,38.05 20.58,39.23 20.59,39.97 v19.67,40.64
  Bottom 0.305: RESET2.1 41.87,50.13 v41.92,50.02 | v31.66,40.37 31.65,40.94 33.45,40.95 34.31,40.97 36.43,40.97 37.1,40.97 37.3,41.2 37.7,41.67 37.7,42.6 v37.11,43.76 | R7.2 20.38,37.92 v20.22,37.44 | U$7.VPP 17.97,46.41 17.98,46.1 18,45.45 18.14,45.3 ATMEGA2.29 | ATMEGA2.29 | ATMEGA2.29 20.2,45.3 20.19,44.36 20.19,41.67 v19.67,40.64
VCC  (via drill 0.5)
  Top 0.305: v4.99,26.98 4.82,27 ATMEGA328.4 4.03,26.98 3.21,26.98 | ATMEGA328.6 7.03,25.4 7.04,25.47 v7.04,26.59 7.03,24.6 ATMEGA328.18 12.61,24.56 12.65,24.56 13.02,24.57 15.04,22.28 15.02,21.34 15.02,6.62 15.04,5.58 2.82,5.6 INTERFACE.1 | R1.1 2.64,30.76 v2.1,30.21 2.08,30.19 2.08,29.19 1.56,28.67 C4.1 | C1.- 14.38,30.48 v14.31,30.46
  Bottom 0.305: 7.09,26.98 v4.99,26.98 2.1,29.99 v2.1,30.21 | 7.09,26.98 7.09,32.72 15.79,32.72 15.79,30.46 | 15.79,30.46 15.78,26.61 15.78,24.83 U$5.VDD | v7.04,26.59 7.09,26.98 | v14.31,30.46 15,30.46 15.79,30.46
VCC1  (via drill 0.5, 0.8)
  Top 0.305: VDD.1 37.96,1.38 37.99,2.08 | 37.16,2.08 37.99,2.08 | ATMEGA1.4 22.81,9.35 | 22.81,9.35 22.79,9.21 22.79,7.91 22.84,7.77 23.84,7.77 ATMEGA1.6 25.32,7.76 26.05,8.37 30.05,8.37 31.46,7.14 31.57,7.03 32.4,7 ATMEGA1.18 33.54,6.91 37.16,6.91 | C3.+ 24.14,15.3 v24.21,15.33 | 37.93,7.83 37.74,7.93 R3.2 37.16,6.91 | R4.2 33.04,14.08 v33,14.04 | 37.99,2.08 37.75,2.38 C2.1 36.4,5.3 v35.68,5.55 36.47,5.28 37.16,5.33 37.51,5.8 37.51,6.52 37.16,6.91 | R2.1 20.84,15.9 20.74,16.03 17.22,16.04 17.23,13.18 17.4,13.2 SENSOR.1 18.7,11.95 20.68,11.79 20.67,9.79 21.04,9.34 22.48,9.35 22.81,9.35 | v45.62,15.05 46.09,15.07 46.1,11.53 INTERFACE1.1
  Bottom 0.305: v33,14.04 24.68,14.04 v24.21,15.33 23.54,15.49 21.83,15.5 22.05,15.09 IC4.VDD 21.97,15.15 21.94,15.18 21.95,16.02 19.13,16.04 17.22,16.03 17.22,13.2 SENSOR.1 | INTERFACE1.1 44.92,11.54 44.92,11.5 44.35,11.5 43.24,10.4 39.88,10.4 39.88,8.66 35.7,8.65 v35.68,5.55
VCC2  (via drill 0.5)
  Top 0.305: RFM69.VDD 30.85,32.37 v30.05,32.31 | v29.11,48.38 29.3,48.47 29.53,49 32.23,48.98 33.19,50.84 33.47,51.31 33.86,51.93 34.93,51.93 43.35,51.93 INTERFACE2.1
  Bottom 0.305: 22.94,33.83 IC3.2 | 25.51,47.35 24.86,45.37 24.04,44.5 24.07,42.45 25.49,41.4 ATMEGA2.18 25.49,39.66 | 25.51,47.35 24.66,48.75 ATMEGA2.6 | ATMEGA2.4 23.09,48.24 24.99,48.26 25.51,47.35 | v29.11,48.38 29.73,47.66 29.96,47.22 29.84,46.66 29.43,46.28 29.41,44.37 30.06,43.99 30.05,43.13 30.04,42.67 30.04,41.35 28.48,41.36 28.48,40.99 28.47,40.11 28.41,40.02 28.05,39.66 | R7.1 23.69,37.87 | IC3.2 | v30.05,32.31 30.24,32.31 | v30.05,32.31 IC3.4 | 29.16,33.73 29.16,33.82 IC3.4 | C11.+ 30.05,30.38 v30.05,32.31 | 28.05,39.66 28.05,37.62 28.48,37.24 28.83,37.07 C12.2 29.13,37.13 IC3.4 | 28.05,39.66 25.49,39.66 | 25.49,39.66 24.33,39.66 24.18,39.5 24.18,38.28 23.69,37.87 | IC3.2 24,33.82 24.47,34.29 24.47,37.09 23.69,37.87

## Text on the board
_tsilk: ANT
